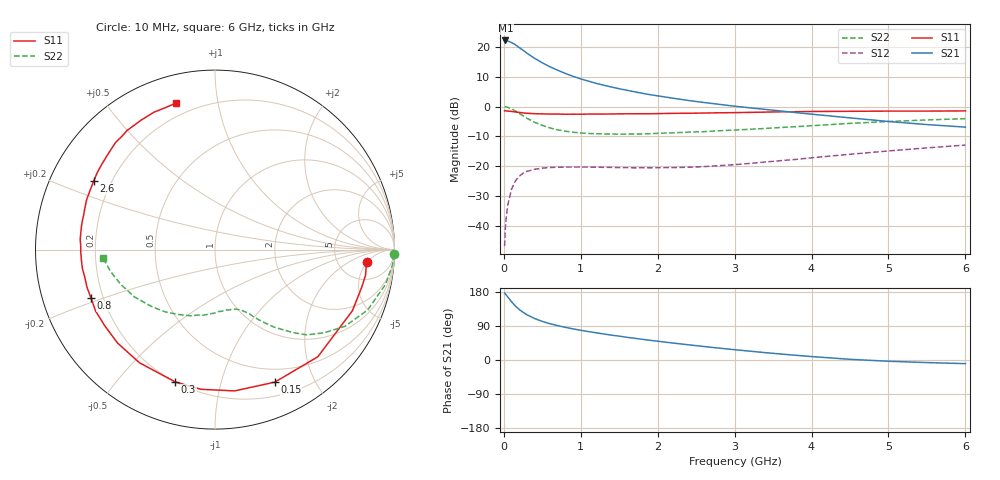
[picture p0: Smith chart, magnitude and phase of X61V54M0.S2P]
! SIEMENS Small Signal Semiconductors
! BFP193W
! Si NPN RF Bipolar Junction Transistor in SOT343
! VCE = 1.5 V  IC = 4 mA
! Common Emitter S-Parameters:  April 1994
# GHz  S  MA  R  50
!  f  S11  S21  S12  S22
! GHz  MAG  ANG  MAG  ANG  MAG  ANG  MAG  ANG
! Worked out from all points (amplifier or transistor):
!   40 points, 10 MHz to 6 GHz, reference 50 ohm
!   highest |S21| = 22.2 dB at 20 MHz (marker M1)
!   |S21| within 3 dB of that: start of sweep to 233.5 MHz
!   unconditionally stable (mu >= 1): 1.746 GHz to 5.544 GHz
!   at 200 MHz: K = 0.12, MSG = 21.6 dB, |S12| = -23.4 dB
!   at 1.5 GHz: K = 0.87, MSG = 13.3 dB, |S12| = -20.5 dB
!   at 6 GHz: K = 0.97, MSG = 3.0 dB, |S12| = -13.0 dB
!   S11 on the Smith chart (normalised r, x): 10 MHz: 10, -5; 150 MHz: 0.35, -1.49; 300 MHz: 0.20, -0.72; 800 MHz: 0.15, -0.18; 2.6 GHz: 0.13, +0.26; 6 GHz: 0.13, +0.76
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0.01  0.8473 -4.8  12.83 176.5  0.0045 88.1  0.9961 -1.5
0.02  0.8508 -9.7  12.88 174.6  0.009 84.7  0.993 -4.8
0.03  0.844 -14.4  12.85 171.9  0.0132 83.3  0.984 -7.0
0.05  0.8379 -24.0  12.65 166.5  0.0218 77.3  0.9699 -11.5
0.1  0.8275 -46.2  11.87 153.9  0.0407 66.5  0.9145 -21.6
0.15  0.8102 -65.7  10.9 142.6  0.0562 56.6  0.8412 -30.5
0.2  0.7949 -82.1  9.78 133.4  0.0673 49.0  0.7648 -37.3
0.25  0.7822 -95.8  8.806 125.9  0.0757 42.7  0.6979 -42.9
0.3  0.7696 -106.8  7.876 119.4  0.0813 37.7  0.6343 -46.8
0.4  0.758 -123.8  6.465 109.5  0.0882 30.4  0.5428 -52.7
0.5  0.7522 -136.2  5.423 101.8  0.0921 25.8  0.4808 -56.7
0.6  0.7466 -145.4  4.643 95.7  0.0944 22.3  0.4364 -59.8
0.8  0.7415 -158.6  3.591 86.1  0.0961 18.5  0.3849 -64.2
1.1  0.7465 -172.0  2.672 75.0  0.0959 16.0  0.3519 -70.4
1.3  0.7479 -178.8  2.274 68.6  0.095 15.8  0.3457 -74.8
1.6  0.7537 172.7  1.874 59.9  0.0939 17.1  0.3437 -81.4
2.2  0.7674 158.8  1.379 44.7  0.0941 23.0  0.3607 -95.4
2.6  0.7767 150.5  1.169 35.6  0.0977 28.2  0.3779 -105.1
3.2  0.796 139.5  0.95 23.3  0.1107 35.0  0.4145 -119.2
4.5  0.8307 119.6  0.644 1.8  0.1575 39.9  0.5207 -149.6
5.5  0.8373 109.7  0.497 -6.8  0.2016 37.0  0.5945 -168.2
6  0.8441 105.1  0.45 -9.6  0.225 34.7  0.6256 -175.7
